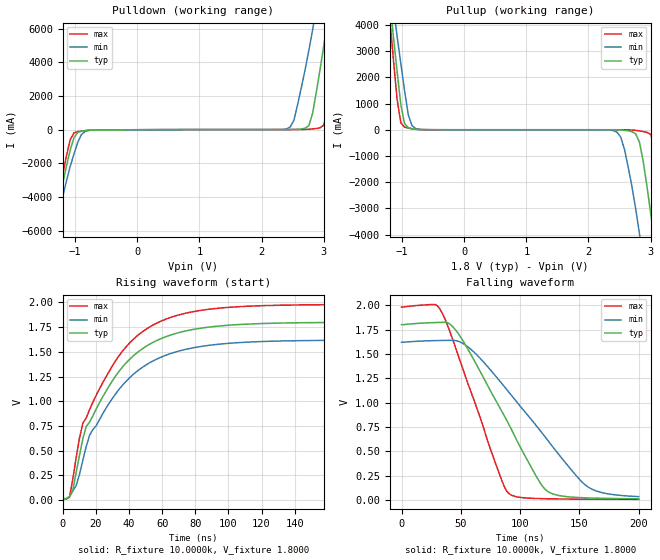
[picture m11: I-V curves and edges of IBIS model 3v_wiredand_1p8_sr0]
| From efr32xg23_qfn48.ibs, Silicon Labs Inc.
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|   Model 3v_wiredand_1p8_sr0
[Model]  3v_wiredand_1p8_sr0
Model_type Output
Polarity   Inverting
Enable   Active-Low
C_comp   1.6300pF   1.4000pF   2.7000pF
[Temperature Range]   25.0000   0.1250k   -40.0000
[Pullup Reference]   1.8000V   1.6200V   1.9800V
[Pulldown Reference]   0.0V   0.0V   0.0V
[POWER Clamp Reference]   1.8000V   1.6200V   1.9800V
[GND Clamp Reference]   0.0V   0.0V   0.0V
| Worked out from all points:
|   slope of the pulldown table from 0 to 0.27 V, typ, clamps not added: 74.9 ohm
|   rising waveform, R_fixture 10.0000k, V_fixture 1.8000: 20-80 % time 32.3ns typ, 33.3ns min, 32.2ns max; typ from 0.011 V to 1.8 V
|   falling waveform, R_fixture 10.0000k, V_fixture 1.8000: 20-80 % time 47ns typ, 63ns min, 33.6ns max; typ from 1.8 V to 0.014 V
[Pulldown]
|Voltage   I(typ)   I(min)   I(max)
-1.8V     -14.24A    -14.11A    -14.46A
-1.38V    -6.469A    -6.98A     -6.162A
-1.14V    -2.142A    -3.024A    -1.536A
-1.02V    -476.1mA   -1.44A     -185.7mA
-780mV    -29.83mA   -36.42mA   -35.11mA
2.46V     11.29mA    161mA      11.75mA
2.76V     243.1mA    4.706A     29.33mA
2.82V     965.9mA    5.915A     48.15mA
2.94V     3.567A     8.549A     112.3mA
3.06V     6.477A     11.36A     1.169A
3.24V     11.26A     15.63A     5.991A
3.6V      20.86A     23.61A     16.8A
[Pullup]
|Voltage   I(typ)   I(min)   I(max)
-1.8V     20.85A     19.71A     22.07A
-1.2V     4.976A     5.911A     4.296A
-1.08V    2.216A     3.565A     1.157A
-960mV    235.8mA    1.496A     100.8mA
-840mV    37.2mA     156.9mA    36.63mA
-720mV    7.125mA    12.82mA    7.666mA
2.46V     -4.689mA   -94.69mA   -342.9uA
2.58V     -21.13mA   -753.1mA   -2.576mA
2.82V     -472.4mA   -3.958A    -43.11mA
3V        -3.168A    -6.98A     -175.3mA
3.24V     -7.604A    -11.14A    -3.782A
3.6V      -14.24A    -16.86A    -10.99A
[Ramp]
| variable   typ   min   max
dV/dt_r  3.1054u/17.7836n   42.4517u/21.4205n   3.2861u/18.6074n
dV/dt_f  1.0718/46.9975n   0.9503/63.0406n   1.1831/33.5870n
R_load = 10.0000k
[Rising Waveform]
R_fixture= 10.0000k
V_fixture= 1.8000
V_fixture_min= 1.6200
V_fixture_max= 1.9800
|time   V(typ)   V(min)   V(max)
0s        11.01mV    16.94mV    7.816mV
4.04ns    37.61mV    33.7mV     28.39mV
6.061ns   101.3mV    92.22mV    215.3mV
12.12ns   620.7mV    404.5mV    778.1mV
16.16ns   789.2mV    654.7mV    914.1mV
20.2ns    922.7mV    752.6mV    1.062V
36.36ns   1.353V     1.168V     1.514V
52.53ns   1.578V     1.39V      1.752V
94.95ns   1.763V     1.579V     1.943V
200ns     1.799V     1.619V     1.979V
[Falling Waveform]
R_fixture= 10.0000k
V_fixture= 1.8000
V_fixture_min= 1.6200
V_fixture_max= 1.9800
|time   V(typ)   V(min)   V(max)
0s        1.8V       1.62V      1.98V
32.32ns   1.823V     1.637V     1.961V
40.4ns    1.81V      1.639V     1.741V
48.48ns   1.698V     1.626V     1.46V
82.83ns   949.2mV    1.222V     258.4mV
90.91ns   767.2mV    1.101V     64.37mV
115.2ns   212.1mV    740.3mV    16.19mV
125.3ns   75.62mV    582mV      13.4mV
157.6ns   22.52mV    132.5mV    9.42mV
200ns     13.6mV     36mV       8.194mV
